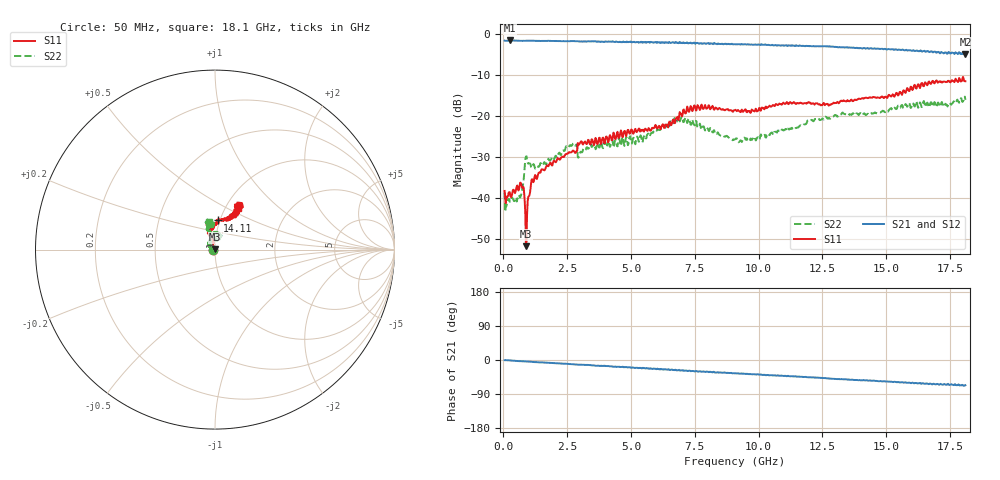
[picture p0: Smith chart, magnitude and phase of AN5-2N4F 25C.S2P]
! Network Analyzer HP8720D.06.14 Serial No. US36140669
! 12 Jan 2005  09:38:32
! Frequency  S11  S21  S12  S22
# HZ  S  DB R 50
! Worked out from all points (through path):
!   801 points, 50 MHz to 18.1 GHz, reference 50 ohm
!   highest |S21| = -1.58 dB at 253.1 MHz (marker M1); lowest = -5.0 dB at 18.1 GHz (marker M2)
!   group delay of S21, straight-line fit = 10.3 ps
!   lowest |S11| = -51.7 dB at 884.8 MHz (marker M3), VSWR 1.01, Z = 49.9 + j0.253 ohm
!   |S11| at or under -10 dB: start of sweep to end of sweep
!   |S22| runs from -43.3 to -15.3 dB; largest |S21 - S12| = 0.028
!   S11 on the Smith chart (normalised r, x): 50 MHz: 0.98, -0.00; 14.11 GHz: 0.98, +0.33; 18.1 GHz: 1.14, +0.57
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5e7  -38.24 -168.0  -1.62 -0.5  -1.62 -0.6  -38.59 -177.5
2.530625e8  -38.55 167.6  -1.58 -1.0  -1.59 -1.5  -40.88 -171.9
6.140625e8  -37.85 140.8  -1.64 -3.0  -1.64 -3.1  -39.21 -172.9
7.26875e8  -37.22 114.0  -1.68 -3.2  -1.65 -3.6  -38.30 -157.0
8.17125e8  -38.90 89.4  -1.67 -3.6  -1.64 -3.8  -34.00 -149.7
8.848125e8  -51.70 103.1  -1.65 -3.7  -1.61 -4.1  -29.90 -171.6
9.525e8  -40.89 170.3  -1.63 -4.1  -1.62 -4.4  -31.34 164.4
1.04275e9  -38.75 155.0  -1.63 -4.4  -1.63 -4.9  -31.55 154.8
1.178125e9  -36.11 142.8  -1.65 -5.4  -1.65 -5.7  -31.70 150.2
2.689812e9  -28.69 105.3  -1.72 -11.1  -1.73 -11.4  -27.17 128.6
3.073375e9  -26.26 98.8  -1.81 -12.7  -1.74 -12.9  -28.85 150.9
5.510125e9  -23.79 103.1  -2.03 -21.7  -2.01 -22.1  -24.99 122.5
6.074188e9  -22.66 108.0  -2.05 -24.2  -2.04 -24.3  -23.35 113.2
6.931562e9  -19.30 105.3  -2.12 -28.1  -2.16 -27.4  -21.02 89.6
7.54075e9  -18.58 94.2  -2.26 -29.1  -2.04 -30.1  -21.18 74.3
9.075e9  -18.55 109.1  -2.51 -34.9  -2.43 -35.2  -25.66 78.9
9.954938e9  -18.80 108.5  -2.59 -37.7  -2.56 -38.5  -25.19 88.5
1.209838e10  -16.96 100.6  -2.98 -46.0  -2.94 -46.3  -21.00 102.7
1.410644e10  -15.75 84.8  -3.47 -53.1  -3.39 -53.7  -19.43 107.2
1.509919e10  -14.84 73.3  -3.68 -57.2  -3.65 -57.1  -18.57 111.2
1.674625e10  -12.15 60.2  -4.24 -62.8  -4.21 -63.9  -16.63 94.7
1.81e10  -11.52 61.0  -4.99 -66.6  -4.97 -69.0  -16.04 102.1
